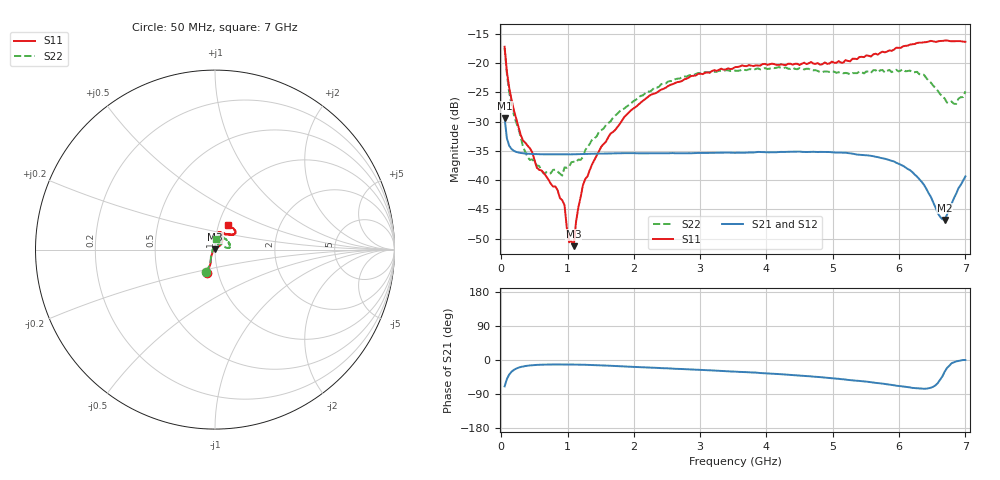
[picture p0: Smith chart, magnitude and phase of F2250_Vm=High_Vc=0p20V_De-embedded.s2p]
! Integrated Device Technology
! Corporate Headquarters
! 6024 Silver Creek Valley Road
! San Jose, CA 95138  USA
! Phone:  1-408-284-8200
! Toll Free:  1-800-223-1366
! Webpage:  http://www.idt.com/
! Timing and RF Division
! 515 Groton Road, Suite 102
! Westford, MA 01886-6024
! Device:  F2250
! Description: Voltage Variable RF Attenuator
! Frequency:  50.0 -  6000.00 MHz
! Package:  3x3 mm Thin QFN Plastic Package: 16 pin
! Ports:  2 RF, 3 DC
!  Pin  1  = GND
!  Pin  2  = NC
!  Pin  3  = RF1  = Port 1
!  Pin  4  = NC
!  Pin  5  = GND
!  Pin  6  = GND
!  Pin  7  = GND
!  Pin  8  = GND
!  Pin  9  = NC
!  Pin 10  = RF2  = Port 2
!  Pin 11  = NC
!  Pin 12  = GND
!  Pin 13  = GND
!  Pin 14  = VCNTRL
!  Pin 15  = VDD
!  Pin 16  = VMODE
! Vcntrl:  0.200 Volts
! Vmode:  +3.300 Volts
! Vdd:  +3.30  Volts
! Current:  1.245 mA
! Data:  The device was measured on a the F2250 evaluation board which has
!  individual transmission lines to the RF pins.  Data was collected
!  using a calibrated network analyzer.  The evaluation board was
!  de-embedded using a TRL calibration technique.
!  The reference plane is the edge of the package pin.
! Misc:  SN 10
!  Action Tracker AT0258
! Date Measured:  2014-11-26
! Date:  2015-10-15  MJV
! Note:
!  Integrated Device Technology supplies this data as a sample of measured
!  data at the package pin for this product.  Your particular data for this
!  product may vary.
!  Data was taken at 25 degrees C.
!  Integrated Device Technology reserves the right to change this data at anytime.
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# GHz S dB R 50
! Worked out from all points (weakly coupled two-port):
!   201 points, 50 MHz to 7 GHz, reference 50 ohm
!   highest |S21| = -29.38 dB at 50 MHz (marker M1); lowest = -46.8 dB at 6.687 GHz (marker M2)
!   lowest |S11| = -51.3 dB at 1.093 GHz (marker M3), VSWR 1.01, Z = 50 + j0.272 ohm
!   |S11| at or under -10 dB: start of sweep to end of sweep
!   |S22| runs from -39.2 to -17.4 dB; largest |S21 - S12| = 5.9e-05
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0.05  -17.18 -108.5  -29.38 -69.5  -29.38 -69.5  -17.37 -110.6
0.08475  -21.47 -107.4  -32.86 -50.1  -32.86 -50.1  -21.87 -109.1
0.15425  -26.23 -116.6  -34.68 -31.0  -34.68 -31.0  -27.10 -120.7
0.29325  -32.27 -127.5  -35.35 -18.5  -35.35 -18.4  -32.66 -133.6
0.3975  -34.12 -142.2  -35.48 -15.0  -35.48 -15.0  -36.08 -158.4
0.5365  -37.87 -154.7  -35.55 -12.9  -35.55 -12.9  -37.50 -179.9
0.64075  -38.79 -162.6  -35.58 -12.2  -35.57 -12.2  -38.88 160.5
0.91875  -43.44 155.9  -35.60 -11.8  -35.60 -11.8  -39.22 127.9
0.9535  -44.25 170.9  -35.60 -11.8  -35.60 -11.8  -37.81 124.3
1.023  -50.63 140.6  -35.59 -11.9  -35.59 -11.9  -37.71 108.1
1.0925  -51.30 89.4  -35.57 -12.0  -35.57 -12.0  -36.85 98.7
1.12725  -47.15 61.8  -35.56 -12.1  -35.56 -12.1  -36.92 91.7
1.2315  -40.85 40.7  -35.53 -12.5  -35.52 -12.5  -36.06 77.2
1.6485  -32.02 41.2  -35.44 -15.2  -35.44 -15.2  -29.92 60.0
2.37825  -24.75 46.7  -35.40 -21.0  -35.40 -21.0  -24.02 53.9
3.525  -20.66 71.8  -35.32 -30.6  -35.32 -30.7  -21.26 72.9
4.7065  -20.06 72.0  -35.15 -43.9  -35.15 -43.9  -21.21 70.3
5.85325  -17.79 40.5  -36.59 -64.8  -36.58 -64.9  -21.13 23.3
6.27025  -16.52 39.4  -39.39 -74.5  -39.40 -74.5  -21.46 8.6
6.68725  -16.11 47.9  -46.80 -31.1  -46.80 -30.7  -26.03 28.5
6.861  -16.22 54.5  -42.32 -3.6  -42.28 -3.7  -26.95 57.5
7  -16.32 62.4  -39.36 -0.1  -39.33 -0.3  -24.81 83.6
